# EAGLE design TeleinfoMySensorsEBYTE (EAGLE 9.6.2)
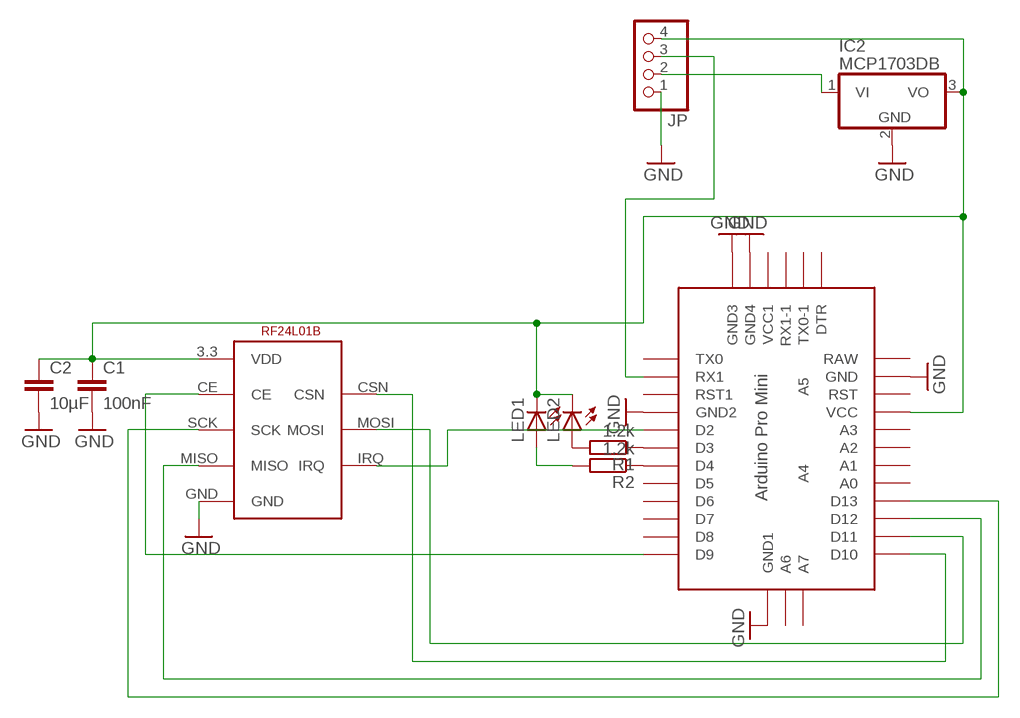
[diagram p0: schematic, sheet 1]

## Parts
C1  100nF  C-EUC1206  [C1206]
C2  10µF  C-EUC1210  [C1210]
IC2  MCP1703DB  [SOT223]
JP  PINHD-1X4  [1X04]
LED1  LED3MM  [LED3MM]
LED2  LED3MM  [LED3MM]
R1  1.2k  R-EU_M1206  [M1206]
R2  1.2k  R-EU_M1206  [M1206]
U$1  ABK-PRO-MINI  [ABK-PRO-MINI]
U$5  NRFL01SMSEBYTE  [24L01SMDEBYTE]

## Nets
GND: C1.2 C2.2 IC2.2(GND) JP.1 U$1.GND U$1.GND1(GND2) U$1.GND2(GND3) U$1.GND3(GND4) U$1.GND4(GND1) U$5.GND
N$1: U$1.D9 U$5.CE
N$2: LED2.A R1.2
N$3: U$1.D13 U$5.SCK
N$4: R1.1 U$1.D3
N$5: IC2.1(VI) JP.2
N$6: U$1.D11 U$5.MOSI
N$7: U$1.D12 U$5.MISO
N$9: R2.1 U$1.D4
N$11: LED1.A R2.2
N$12: JP.3 U$1.RX1
N$14: C1.1 C2.1 IC2.3(VO) JP.4 LED1.K(C) LED2.K(C) U$1.VCC U$5.3.3(VDD)
N$18: U$1.D2 U$5.IRQ
N$19: U$1.D10 U$5.CSN
Unconnected: U$1.A0 U$1.A1 U$1.A2 U$1.A3 U$1.A4 U$1.A5 U$1.A6 U$1.A7 U$1.D5 U$1.D6 U$1.D7 U$1.D8 U$1.DTR U$1.RAW U$1.RST U$1.RST1 U$1.RX1-1 U$1.TX0 U$1.TX0-1 U$1.VCC1

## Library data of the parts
C1 C2 = rcl:C-EU: CAPACITOR, European symbol
IC2 = linear:MCP1703: 250 mA, 16V, Low Quiescent Current LDO Regulator Source: http://ww1.microchip.com/downloads/en/DeviceDoc/22049b.pdf
JP = pinhead:PINHD-1X4: PIN HEADER
LED1 LED2 = led:LED: LED
R1 R2 = rcl:R-EU_: RESISTOR, European symbol
U$1 = Arduino-clone:ABK-PRO-MINI: ABK Pro-Mini Arduino Clone
U$5 = nrf24l01:NRFL01SMSEBYTE

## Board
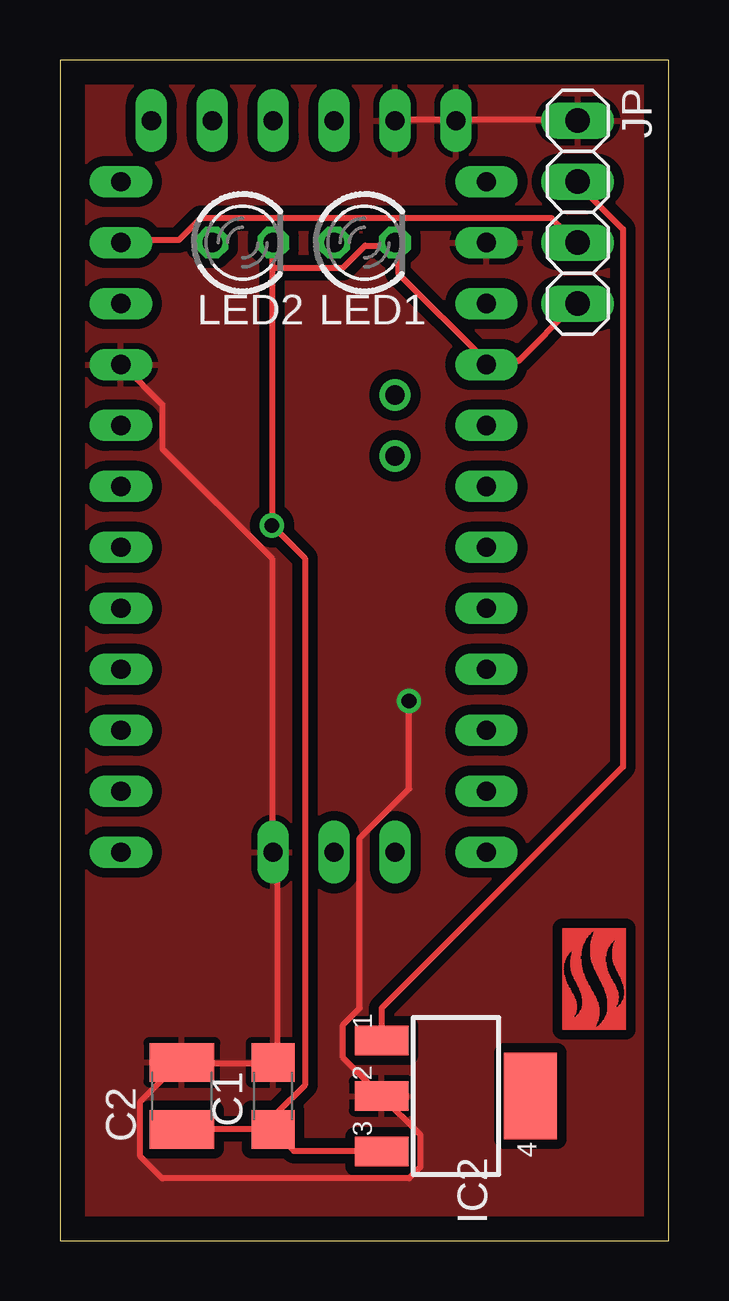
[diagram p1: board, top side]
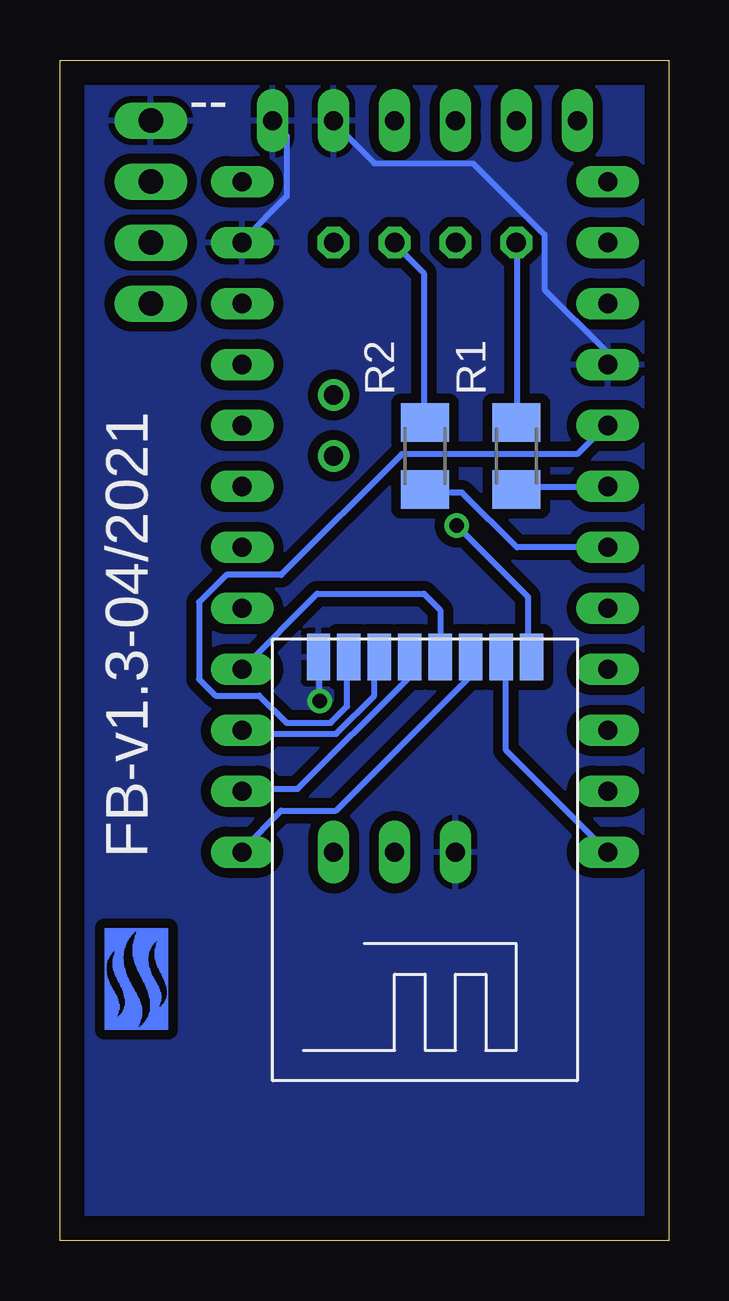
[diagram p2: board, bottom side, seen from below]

Size 25.38 x 49.2 mm. Coordinates in mm from the lower left corner, seen from the top.
Outline: 0,0 25.38,0 25.38,49.2 0,49.2 0,0
Copper layers (1*16): Top 0.035mm / dielectric 1.5mm / Bottom 0.035mm
Design rules "default": minimum track width 10mil, minimum drill 24mil, track to track 8mil, track to pad 8mil, pad to pad 8mil, via to via 8mil, smd to smd 8mil, copper to edge 40mil, drill to drill 8mil, minimum pad ring 10mil, minimum via ring 8mil, stop-mask expansion 4mil, vias tented up to drill 0mil, thermal gap 10mil

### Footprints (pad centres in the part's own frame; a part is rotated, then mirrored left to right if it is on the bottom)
C1206 = smd 1.6 x 1.8: 1 -1.4,0; 2 1.4,0
C1210 = smd 1.6 x 2.7: 1 -1.4,0; 2 1.4,0
SOT223 = smd 1.219 x 2.235: 1 -2.311,-3.099; 2 0,-3.099; 3 2.311,-3.099 | smd 3.6 x 2.2: 4 0,3.099
1X04 = drill 1.016 long: 1 -3.81,0; 2 -1.27,0; 3 1.27,0; 4 3.81,0
LED3MM = drill 0.813 octagon: A -1.27,0; K 1.27,0
M1206 = smd 1.6 x 2: 1 -1.4,0; 2 1.4,0
ABK-PRO-MINI = drill 0.8 long: A0 10.16,-11.43; A1 10.16,-8.89; A2 10.16,-6.35; A3 10.16,-3.81; A6 3.81,-21.59; A7 6.35,-21.59; D2 -5.08,-3.81; D3 -5.08,-6.35; D4 -5.08,-8.89; D5 -5.08,-11.43; D6 -5.08,-13.97; D7 -5.08,-16.51; D8 -5.08,-19.05; D9 -5.08,-21.59; D10 10.16,-21.59; D11 10.16,-19.05; D12 10.16,-16.51; D13 10.16,-13.97; DTR -3.81,8.89; GND 10.16,3.81; GND1 -5.08,-1.27; GND2 8.89,8.89; GND3 6.35,8.89; GND4 1.27,-21.59; RAW 10.16,6.35; RST 10.16,1.27; RST1 -5.08,1.27; RX1 -5.08,3.81; RX1-1 1.27,8.89; TX0 -5.08,6.35; TX0-1 -1.27,8.89; VCC 10.16,-1.27; VCC1 3.81,8.89 | drill 0.8: A4 6.35,-5.08; A5 6.35,-2.54
24L01SMDEBYTE = smd 1.93 x 0.965: 3.3 -8.128,4.445; CE -8.128,3.175; CSN -8.128,1.905; GND -8.128,-4.445; IRQ -8.128,-3.175; MISO -8.128,-1.905; MOSI -8.128,-0.635; SCK -8.128,0.635

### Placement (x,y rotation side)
C1  8.89,6.03 90 top
C2  5.08,6.03 90 top
IC2  16.51,6.03 270 top
JP  21.59,42.86 270 top
LED1  12.7,41.59 0 top
LED2  7.62,41.59 0 top
R1  6.35,32.7 90 bottom
R2  10.16,32.7 90 bottom
U$1  7.62,37.78 0 top
U$3  [FB]  23.49,13.02 180 top
U$4  [FB]  20.95,13.02 180 bottom
U$5  10.16,16.19 270 bottom

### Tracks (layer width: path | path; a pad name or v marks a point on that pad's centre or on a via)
GND  (via drill 0.61)
  Top 0.254: v14.55,22.49 14.55,18.83 12.5,16.78 12.5,9.69 11.81,9 11.81,7.63 IC2.2 15.01,4.43 15.01,3.06 14.55,2.6 4.27,2.6 3.35,3.52 3.35,5.8 4.95,7.4 C2.2 5.18,7.4 8.84,7.4 C1.2 9.07,7.63 9.07,16.09 U$1.GND4 8.84,16.32 8.84,28.44 4.27,33.01 4.27,34.84 2.67,36.44 U$1.GND1 | U$1.GND3 14.1,46.72 16.38,46.72 U$1.GND2 16.61,46.72 21.41,46.72 JP.1
  Bottom 0.254: v14.55,22.49 14.55,24.32 U$5.GND | U$1.GND1 2.67,36.66 2.67,37.12 5.18,39.64 5.18,41.92 8.15,44.89 12.27,44.89 13.87,46.49 U$1.GND3 | U$1.GND 17.75,41.69 15.93,43.52 15.93,46.04 16.38,46.49 U$1.GND2
  pour Top (isolate 0.406): 0,49.21 25.4,49.21 25.4,-0.32 0,-0.32
  pour Bottom (isolate 0.406): 0,49.21 25.4,49.21 25.4,-0.32 0,-0.32
N$1
  Bottom 0.254: U$1.D9 6.78,20.43 6.78,24.32 U$5.CE
N$2
  Bottom 0.254: R1.2 6.33,34.15 6.33,41.47 LED2.A
N$3
  Bottom 0.254: U$5.SCK 9.53,26.28 10.21,26.96 14.66,26.96 17.75,23.86 U$1.D13
N$4
  Bottom 0.254: R1.1 6.33,31.41 2.67,31.41 U$1.D3
N$5
  Top 0.254: IC2.1 13.41,9.69 23.47,19.75 23.47,42.15 21.64,43.98 JP.2
N$6
  Bottom 0.254: U$5.MOSI 10.9,24.32 10.9,23.41 15.47,18.83 17.75,18.83 U$1.D11
N$7
  Bottom 0.254: U$5.MISO 12.27,24.32 12.27,22.72 13.87,21.12 17.75,21.12 U$1.D12
N$9
  Bottom 0.254: U$1.D4 6.33,28.89 8.61,31.18 9.98,31.18 R2.1
N$11
  Bottom 0.254: R2.2 10.21,34.15 10.21,40.32 11.35,41.47 LED1.A
N$12
  Top 0.254: U$1.RX1 2.67,41.69 4.95,41.69 5.87,42.61 20.5,42.61 21.41,41.69 JP.3
N$14  (via drill 0.61)
  Top 0.254: C1.1 8.84,4.66 5.18,4.66 C2.1 | IC2.3 13.41,3.75 9.75,3.75 9.07,4.43 C1.1 | JP.4 21.41,38.95 19.13,36.66 17.98,36.66 U$1.VCC 17.75,36.66 14.1,40.32 14.1,41.47 LED1.K 13.87,41.47 12.72,41.47 11.81,40.55 8.84,40.55 | 8.84,40.55 8.84,41.47 LED2.K | 8.84,40.55 v8.84,29.81 10.21,28.44 10.21,6.49 9.07,5.35 9.07,4.66 C1.1
  Bottom 0.254: v8.84,29.81 5.87,26.84 5.87,24.32 U$5.3.3
N$18
  Bottom 0.254: U$5.IRQ 13.41,24.32 13.41,22.26 14.1,21.58 15.93,21.58 17.07,22.72 18.9,22.72 19.58,23.41 19.58,26.61 18.44,27.75 16.15,27.75 11.12,32.78 3.81,32.78 2.67,33.92 U$1.D2
N$19
  Bottom 0.254: U$5.CSN 8.38,24.32 8.38,23.41 13.87,17.92 16.15,17.92 17.75,16.32 U$1.D10

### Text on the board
bNames: -- | FB-v1.3-04/2021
